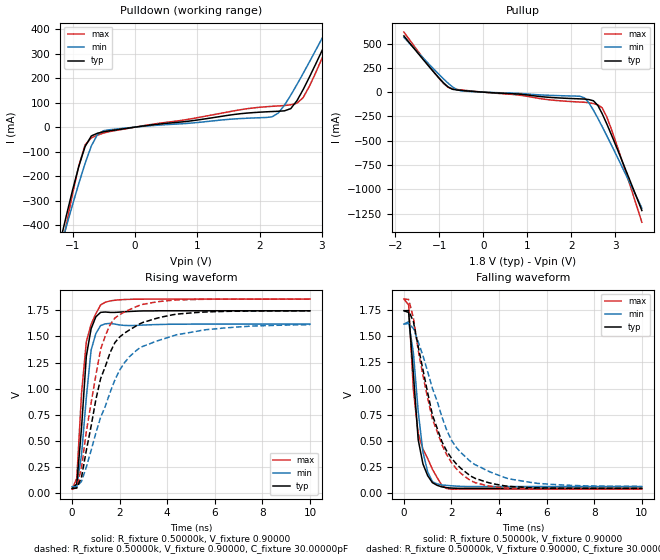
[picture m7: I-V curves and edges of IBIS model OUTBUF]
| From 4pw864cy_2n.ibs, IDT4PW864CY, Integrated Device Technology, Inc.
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|   Model OUTBUF
[Model]   OUTBUF
Model_type   Output
Polarity   Inverting
Vmeas =  0.90000V
C_comp   6.50000pF   5.40000pF   8.10000pF
[Temperature Range]   25.00000   0.11000k   0.000
[Voltage Range]   1.80000V   1.70000V   1.90000V
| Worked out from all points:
|   slope of the pulldown table from 0 to 0.27 V, typ, clamps not added: 29.7 ohm
|   slope of the pullup table from 0 to 0.27 V, typ, clamps not added: 35.5 ohm
|   rising waveform, R_fixture 0.50000k, V_fixture 0.90000: 20-80 % time 363ps typ, 372ps min, 391ps max; typ from 0.047 V to 1.74 V
|   rising waveform, R_fixture 0.50000k, V_fixture 0.90000, C_fixture 30.00000pF: 20-80 % time 1.14ns typ, 1.65ns min, 888ps max; typ from 0.047 V to 1.74 V
|   falling waveform, R_fixture 0.50000k, V_fixture 0.90000: 20-80 % time 400ps typ, 408ps min, 567ps max; typ from 1.74 V to 0.047 V
|   falling waveform, R_fixture 0.50000k, V_fixture 0.90000, C_fixture 30.00000pF: 20-80 % time 1.25ns typ, 1.65ns min, 1.21ns max; typ from 1.74 V to 0.047 V
[Pulldown]
| voltage   I(typ)   I(min)   I(max)
-1.8V     -1.143A    -1.055A    -1.369A
-1.2V     -468.2mA   -494.8mA   -530.4mA
-1.1V     -360.3mA   -404.2mA   -397.3mA
-900mV    -159.4mA   -229.2mA   -157.4mA
-700mV    -35.92mA   -76.98mA   -43.85mA
-500mV    -18.76mA   -14.23mA   -23.74mA
2.2V      63.59mA    42.02mA    84.92mA
2.5V      75.54mA    130.3mA    91.16mA
2.7V      153.8mA    219.6mA    120.8mA
3.1V      365.6mA    409.3mA    339.1mA
3.2V      420.7mA    457.7mA    399.4mA
3.6V      644mA      653.4mA    645.3mA
[Pullup]
| voltage   I(typ)   I(min)   I(max)
-1.8V     578.2mA    563.7mA    617.9mA
-1.1V     194.8mA    227mA      195.6mA
-800mV    54.3mA     93.41mA    50.68mA
-500mV    17.9mA     13.27mA    22.79mA
2.2V      -69.13mA   -43.15mA   -102mA
2.3V      -71.41mA   -59.75mA   -104.4mA
2.5V      -88.66mA   -184.8mA   -118mA
2.6V      -135.6mA   -267.6mA   -130.6mA
2.7V      -221.8mA   -354.8mA   -161.5mA
2.8V      -322.5mA   -444.4mA   -250.6mA
3V        -538.3mA   -627.8mA   -500.9mA
3.6V      -1.218A    -1.192A    -1.338A
[Ramp]
| variable   typ   min   max
dV/dt_r   1.01160/0.36749n   0.91800/0.40190n   1.08660/0.40642n
dV/dt_f   1.02281/0.40583n   0.94146/0.44243n   1.09082/0.59566n
R_load = 0.50000k
[Rising Waveform]
R_fixture = 0.50000k
V_fixture = 0.90000
V_fixture_min = 0.85000
V_fixture_max = 0.95000
| time   V(typ)   V(min)   V(max)
0s        46.99mV    63.92mV    40.56mV
200ps     90.65mV    69.19mV    145mV
400ps     631.7mV    372.1mV    960.2mV
600ps     1.31V      916.3mV    1.447V
800ps     1.572V     1.368V     1.615V
1ns       1.686V     1.527V     1.716V
1.2ns     1.729V     1.603V     1.8V
1.6ns     1.728V     1.623V     1.838V
2.4ns     1.738V     1.603V     1.853V
10ns      1.744V     1.617V     1.856V
[Rising Waveform]
R_fixture = 0.50000k
V_fixture = 0.90000
V_fixture_min = 0.85000
V_fixture_max = 0.95000
C_fixture = 30.00000pF
| time   V(typ)   V(min)   V(max)
0s        46.99mV    63.92mV    40.56mV
200ps     51.47mV    62.57mV    55.12mV
400ps     157.3mV    116.6mV    249.8mV
600ps     410mV      251.7mV    589.8mV
1.2ns     1.096V     726.2mV    1.376V
1.8ns     1.44V      1.083V     1.675V
2.2ns     1.53V      1.247V     1.732V
2.8ns     1.615V     1.383V     1.793V
4.4ns     1.712V     1.516V     1.847V
10ns      1.744V     1.612V     1.856V
[Falling Waveform]
R_fixture = 0.50000k
V_fixture = 0.90000
V_fixture_min = 0.85000
V_fixture_max = 0.95000
| time   V(typ)   V(min)   V(max)
0s        1.744V     1.617V     1.856V
200ps     1.728V     1.639V     1.8V
400ps     1.138V     1.341V     984.9mV
600ps     513.6mV    783.1mV    570.8mV
800ps     280.6mV    394.2mV    422.8mV
1ns       167.9mV    203.6mV    331.3mV
1.2ns     100.7mV    109.8mV    229.1mV
1.6ns     60.26mV    78.92mV    74.04mV
2ns       49.62mV    71.47mV    39.17mV
10ns      46.99mV    63.92mV    40.56mV
[Falling Waveform]
R_fixture = 0.50000k
V_fixture = 0.90000
V_fixture_min = 0.85000
V_fixture_max = 0.95000
C_fixture = 30.00000pF
| time   V(typ)   V(min)   V(max)
0s        1.744V     1.617V     1.856V
200ps     1.746V     1.623V     1.852V
400ps     1.64V      1.575V     1.675V
800ps     1.182V     1.316V     1.126V
1.2ns     747mV      1.001V     706.6mV
1.8ns     402.7mV    602.9mV    367.9mV
2.4ns     237.1mV    387.4mV    189mV
3ns       141.7mV    271.8mV    101.1mV
4.4ns     66.12mV    138.6mV    48.42mV
10ns      47.03mV    65.14mV    40.56mV
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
